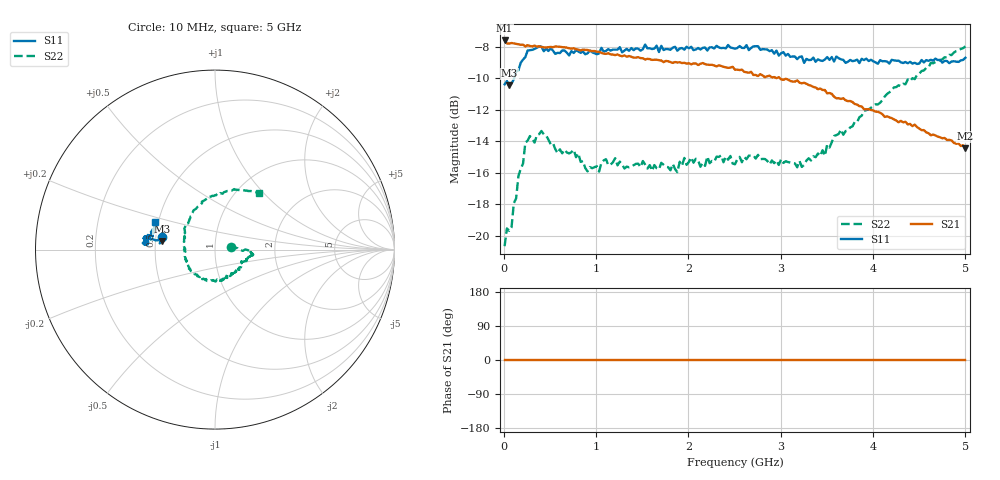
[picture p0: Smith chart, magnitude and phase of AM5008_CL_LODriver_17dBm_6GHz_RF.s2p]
!Keysight Technologies,N5245B,MY58422270,A.16.20.02
!Mixer S2P File: Scalar Mixer Measurement
!Calibration State: On
!Parameters: Stimulus Freq, S11, SC21, SC12, S22
# Hz  S  DB  R  50.0
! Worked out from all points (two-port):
!   201 points, 10 MHz to 5 GHz, reference 50 ohm
!   highest |S21| = -7.61 dB at 10 MHz (marker M1); lowest = -14.5 dB at 5 GHz (marker M2)
!   |S21| within 3 dB of the highest: start of sweep to 3.382 GHz
!   lowest |S11| = -10.5 dB at 59.9 MHz (marker M3), VSWR 1.86, Z = 27 + j2.9 ohm
!   |S11| at or under -10 dB: start of sweep to 112.9 MHz
!   |S22| runs from -20.6 to -8.0 dB; largest |S21 - S12| = 0.42
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1e7  -10.39 166.1  -7.61 0.0  -200.00 90.0  -20.65 8.7
3.495e7  -10.18 173.7  -7.80 0.0  -200.00 90.0  -19.52 3.1
5.99e7  -10.45 170.6  -7.81 0.0  -200.00 90.0  -19.68 3.1
8.485e7  -10.35 169.2  -7.77 0.0  -200.00 90.0  -19.46 7.1
2.3455e8  -8.66 170.7  -7.98 0.0  -200.00 90.0  -14.09 -2.3
2.8445e8  -8.22 171.1  -7.96 0.0  -200.00 90.0  -13.67 -4.4
4.092e8  -8.00 171.5  -8.02 0.0  -200.00 90.0  -13.35 -7.4
5.8385e8  -8.39 173.1  -8.00 0.0  -200.00 90.0  -14.75 -14.2
8.583e8  -8.30 174.9  -8.18 0.0  -200.00 90.0  -15.25 -22.7
9.082e8  -8.42 175.2  -8.21 0.0  -200.00 90.0  -15.91 -24.4
1.2076e9  -8.19 174.4  -8.54 0.0  -200.00 90.0  -15.07 -39.5
1.68165e9  -8.34 174.0  -8.85 0.0  -200.00 90.0  -15.78 -56.1
2.2056e9  -8.25 172.2  -9.14 0.0  -200.00 90.0  -14.97 -89.0
2.505e9  -8.13 171.6  -9.46 0.0  -200.00 90.0  -15.45 -119.6
2.7545e9  -7.97 169.9  -9.86 0.0  -200.00 90.0  -14.86 -143.6
3.17865e9  -8.79 167.5  -10.14 0.0  -200.00 90.0  -15.65 -175.9
3.3533e9  -8.69 166.8  -10.55 0.0  -200.00 90.0  -14.95 165.7
3.47805e9  -8.81 166.3  -10.75 0.0  -200.00 90.0  -14.92 153.9
3.6527e9  -8.80 164.4  -11.31 0.0  -200.00 90.0  -13.25 138.3
4.17665e9  -9.07 160.3  -12.48 0.0  -200.00 90.0  -10.90 100.1
4.62575e9  -8.83 156.8  -13.62 0.0  -200.00 90.0  -9.03 72.4
5e9  -8.71 155.2  -14.45 0.0  -200.00 90.0  -7.98 52.5
